PROGRAM MAIN
VAR
	fbVisus						: FB_Visus;
	
	bStart						: BOOL		:=TRUE;
	bStop						: BOOL;
	bReset						: BOOL;
	
	// 对象实例
	fbShowMotion				: FB_ShowMotion;	
	
	// 接口
	iShowMotion					: I_ShowMotion			:= fbShowMotion;
	iShowRuntime				: I_Runtime				:= fbShowMotion;
	iVisusRuntime				: I_Runtime				:= fbVisus;
END_VAR

iShowRuntime.Cyclic();

// 设置运动方式

iShowMotion.ShowPattern	:= 2;

// 启动
IF bStart THEN
	iShowMotion.P_Start	:= TRUE;
	bStart:= FALSE;
END_IF
IF bStop THEN
	iShowMotion.P_Stop	:= TRUE;
	 bStop:= FALSE;
END_IF
IF bReset THEN
	iShowMotion.P_Reset	:= TRUE;
	bReset	:= FALSE;
END_IF

// HMI
iVisusRuntime.Cyclic();

END_PROGRAM
